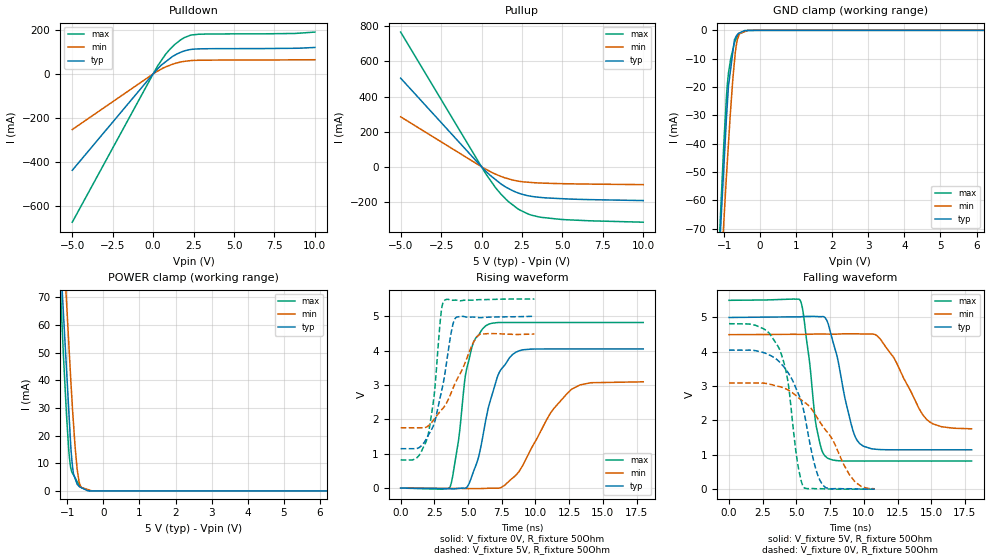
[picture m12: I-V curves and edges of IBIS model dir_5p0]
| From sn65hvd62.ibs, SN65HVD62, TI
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|   dir_5p0 Model
[Model]   dir_5p0
Model_type   3-state
Polarity   Non-Inverting
Vmeas = 2.5
Vref = 2.5
Cref = 2pF
Rref = 50
|   typ   min   max
|   (nom PVT)   (fast PVT)   (slow PVT)
 C_comp   2.572e-12   2.386e-12   2.994e-12
|ON state : BUFFER OUTPUT TURNED HIGH
C_comp   2.572e-12   2.386e-12   2.994e-12
|OFF state: BUFFER IN HIGH IMPEDANCE
|C_comp   1.451e-12   1.431e-12   1.472e-12
| Where nom  PVT is Nominal Process, 5V, 27C
|   Fast PVT is Strong Process,  5.5V, -40C
|   Slow PVT is Weak Process,   4.5V, 125C
[Voltage Range]   5   4.5   5.5
|Ambient Temperature   25   85   -40
|Junction Temperature
[Temperature Range]   27   125   -40
[Pullup Reference]   5   4.5   5.5
[Pulldown Reference]   0   0   0
[Power Clamp Reference]   5   4.5   5.5
[GND Clamp Reference]   0   0   0
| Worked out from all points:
|   slope of the pulldown table from 0 to 0.75 V, typ, clamps not added: 13.9 ohm
|   slope of the pullup table from 0 to 0.75 V, typ, clamps not added: 11.6 ohm
|   GND clamp passes 1 mA (typ) near -0.59 V on its own axis
|   POWER clamp passes 1 mA (typ) near -0.58 V on its own axis
|   falling waveform, V_fixture 5V, R_fixture 50Ohm: 20-80 % time 1.29ns typ, 2.16ns min, 825ps max; typ from 5 V to 1.15 V
|   rising waveform, V_fixture 0V, R_fixture 50Ohm: 20-80 % time 1.47ns typ, 2.72ns min, 1.02ns max; typ from 0 V to 4.05 V
|   rising waveform, V_fixture 5V, R_fixture 50Ohm: 20-80 % time 1.1ns typ, 1.97ns min, 736ps max; typ from 1.15 V to 5 V
|   falling waveform, V_fixture 0V, R_fixture 50Ohm: 20-80 % time 1.67ns typ, 2.85ns min, 1.07ns max; typ from 4.05 V to 0.001 V
[Pulldown]
|   Voltage   I(typ)   I(min)   I(max)
-5V       -438.6mA   -253.1mA   -674.8mA
264mV     22.33mA    12.16mA    34.71mA
759mV     54.5mA     31.39mA    88.1mA
968mV     66.36mA    37.48mA    106.6mA
1.205V    79.8mA     44.23mA    124.2mA
1.672V    97.49mA    53.47mA    153.5mA
2.316V    111.1mA    60.41mA    176.3mA
2.8V      113.9mA    62.11mA    180.4mA
8.794V    116.7mA    64.08mA    184.2mA
10V       120.5mA    64.58mA    190.3mA
[GND Clamp]
|   Voltage   I(typ)   I(min)   I(max)
-5V       -1.334A    -1.212A    -1.473A
-1.14V    -80.79mA   -98.91mA   -76.74mA
-1.105V   -71.85mA   -90.48mA   -66.53mA
-1.062V   -61.32mA   -79.9mA    -54.7mA
-1.006V   -48.01mA   -67.42mA   -39.7mA
-907.5mV  -25.31mA   -45.78mA   -18.72mA
-880mV    -19.76mA   -40.12mA   -15.19mA
-756mV    -7.449mA   -16.88mA   -6.734mA
-715mV    -3.378mA   -11.26mA   -4.542mA
-634.5mV  -1.538mA   -3.319mA   -2.097mA
-435mV    -87.47uA   -468.1uA   -466.5uA
10V       0A         0A         0A
[Pullup]
|   Voltage   I(typ)   I(min)   I(max)
-5V       504.5mA    284.4mA    766.8mA
280.5mV   -26.66mA   -14.77mA   -42.41mA
968mV     -80.49mA   -45.9mA    -130.6mA
1.672V    -124mA     -68.92mA   -198.9mA
2.376V    -152.9mA   -83.53mA   -246.6mA
2.909V    -165.5mA   -88.34mA   -270mA
3.691V    -175mA     -92.77mA   -287.9mA
5.192V    -182.7mA   -96.61mA   -301.4mA
10V       -192.5mA   -101.8mA   -315.6mA
[POWER Clamp]
|   Voltage   I(typ)   I(min)   I(max)
-5V       1.265A     1.219A     1.33A
-1.373V   135mA      158.6mA    123.9mA
-1.14V    71.46mA    97.91mA    57.76mA
-1.062V   53.04mA    77.57mA    37.1mA
-1.023V   43.82mA    68.26mA    27.29mA
-951.5mV  26.94mA    51.18mA    13.15mA
-900mV    15.07mA    38.88mA    8.002mA
-830mV    6.102mA    24.31mA    5.749mA
-733.5mV  2.656mA    8.445mA    3.486mA
-679.5mV  1.703mA    3.644mA    2.219mA
-435mV    48.38uA    512.5uA    255.2uA
10V       0A         0A         0A
[Ramp]
R_load = 50
|   typ   min   max
dV/dt_r   2.42899/1.46429e-09   1.8551/2.74057e-09   2.8916/1.02471e-09
dV/dt_f   2.31251/1.28996e-09   1.64512/2.14224e-09   2.8087/8.22926e-10
[Falling Waveform]
V_fixture = 5V
V_fixture_min = 4.5V
V_fixture_max = 5.5V
R_fixture = 50Ohm
|   Time   V(typ)   V(min)   V(max)
0s        5V         4.5V       5.5V
5.272ns   5.019V     4.509V     5.505V
5.944ns   5.031V     4.511V     3.797V
6.468ns   5.029V     4.517V     1.835V
7.284ns   4.888V     4.516V     911.1mV
9.04ns    1.926V     4.525V     818.7mV
9.7ns     1.326V     4.521V     818.6mV
11.19ns   1.154V     4.386V     818.8mV
14.66ns   1.146V     2.029V     818.8mV
18ns      1.146V     1.758V     818.8mV
[Rising Waveform]
V_fixture = 0V
V_fixture_min = 0V
V_fixture_max = 0V
R_fixture = 50Ohm
|   Time   V(typ)   V(min)   V(max)
0s        4.801nV    26.21nV    3.497nV
3.66ns    -20.62mV   -10.77mV   29.9mV
4.284ns   -10.13mV   -10.03mV   1.362V
4.884ns   13.86mV    -15.5mV    3.446V
5.74ns    845.6mV    -15.34mV   4.438V
6.308ns   1.968V     -8.858mV   4.721V
7.22ns    3.283V     -2.409mV   4.817V
8.524ns   3.948V     364mV      4.819V
12.7ns    4.048V     2.879V     4.819V
18ns      4.048V     3.092V     4.819V
[Rising Waveform]
V_fixture = 5V
V_fixture_min = 4.5V
V_fixture_max = 5.5V
R_fixture = 50Ohm
|   Time   V(typ)   V(min)   V(max)
0s        1.146V     1.754V     818.8mV
1.196ns   1.148V     1.754V     879.9mV
1.984ns   1.491V     1.791V     1.46V
2.488ns   1.879V     2.004V     2.708V
2.944ns   2.661V     2.234V     4.89V
3.188ns   3.111V     2.346V     5.433V
3.812ns   4.653V     2.835V     5.464V
4.14ns    4.972V     3.133V     5.47V
5.828ns   4.957V     4.464V     5.482V
9.92ns    4.999V     4.482V     5.5V
[Falling Waveform]
V_fixture = 0V
V_fixture_min = 0V
V_fixture_max = 0V
R_fixture = 50Ohm
|   Time   V(typ)   V(min)   V(max)
0s        4.048V     3.092V     4.819V
2.508ns   3.984V     3.091V     4.681V
3.732ns   3.709V     2.987V     4.087V
4.324ns   3.425V     2.901V     3.24V
5.072ns   2.844V     2.69V      789.5mV
5.58ns    2.218V     2.537V     37.71mV
6.28ns    819.6mV    2.246V     16.56mV
6.956ns   122.3mV    1.831V     10.87mV
9.368ns   7.513mV    203.6mV    -41.44uV
10.81ns   575.8uV    11.35mV    -472.2nV
